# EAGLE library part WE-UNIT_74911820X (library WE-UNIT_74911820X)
Off-Line Transformer WE-Unit - Nominal input voltage: 85-265 VAC - Output power 9 W - Operating temperature: -40°C to +125 °C - Clearance and creepage distance 6 mm min. - Isolation voltage 4 kVAC -- Designed for Tiny switch ICs from power integration and NCP101x or 105x of Semiconductor -- Universal input -- Offline-switch mode power supplies
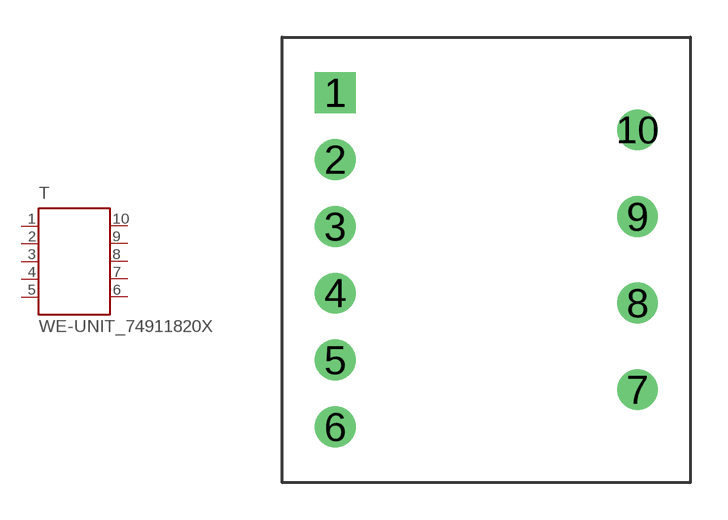
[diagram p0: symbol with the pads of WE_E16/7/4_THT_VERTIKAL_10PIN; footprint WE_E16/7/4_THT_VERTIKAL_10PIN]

Designator prefix T

## WE-UNIT_74911820X, WE-UNIT_74911820X-7491182012 (MPN: 7491182012; OC_FARNELL: 1849036; OC_NEWARK: 13T9797; PACKAGE: E16_7_4; SUPPLIER: Wuerth Elektronik), WE-UNIT_74911820X-7491182024 (MPN: 7491182024; OC_FARNELL: 1849038; OC_NEWARK: 13T9798; PACKAGE: E16_7_4; SUPPLIER: Wuerth Elektronik), WE-UNIT_74911820X-749118205 (MPN: 749118205; OC_FARNELL: 1849035; OC_NEWARK: 13T9799; PACKAGE: E16_7_4; SUPPLIER: Wuerth Elektronik)  [WE_E16/7/4_THT_VERTIKAL_10PIN]
1  1  pas
2  2  pas
3  3  pas
4  4  pas
5  5  pas
6  6  pas
7  7  pas
8  8  pas
9  9  pas
10  10  pas

## Footprint WE_E16/7/4_THT_VERTIKAL_10PIN (pad centres in mm)
Transformer, E16/7/4 THT Vertikal 10 Pin
drill 1.1 square: 1 -6.1,6.75
drill 1.1: 2 -6.1,4.05; 3 -6.1,1.35; 4 -6.1,-1.35; 5 -6.1,-4.05; 6 -6.1,-6.75; 7 6.1,-5.25; 8 6.1,-1.75; 9 6.1,1.75; 10 6.1,5.25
